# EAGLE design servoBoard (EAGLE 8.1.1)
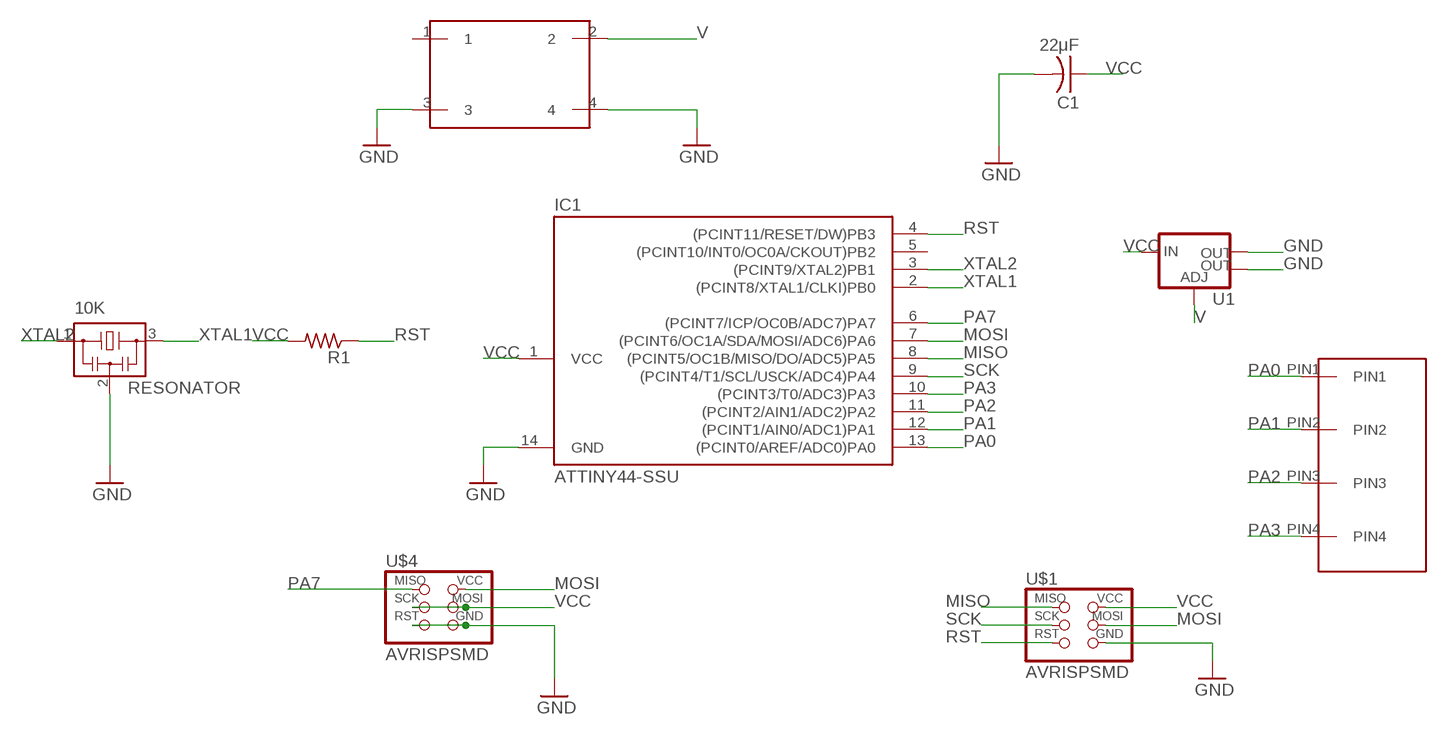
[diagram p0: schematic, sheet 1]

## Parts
10K  RESONATOR  [EFOBM]
C1  22μF  CAP-US1206FAB  [C1206FAB]
IC1  ATTINY44-SSU  [SOIC14]
R1  RES-US1206FAB  [R1206FAB]
U1  V_REG_LM1117SOT223  [SOT223]
U$1  AVRISPSMD  [2X03SMD]
U$2  4PINHEADER2X2  [2X02SMD]
U$3  4PINHEADER_ALTERNATE  [4PINHEADER]
U$4  AVRISPSMD  [2X03SMD]

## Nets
GND: 10K.2 C1.2 IC1.14(GND) U1.2(OUT) U1.4(OUT) U$1.6(GND) U$2.3 U$2.4 U$4.5(RST) U$4.6(GND)
MISO: IC1.8((PCINT5/OC1B/MISO/DO/ADC5)PA5) U$1.1(MISO)
MOSI: IC1.7((PCINT6/OC1A/SDA/MOSI/ADC6)PA6) U$1.4(MOSI) U$4.2(VCC)
PA0: IC1.13((PCINT0/AREF/ADC0)PA0) U$3.PIN1
PA1: IC1.12((PCINT1/AIN0/ADC1)PA1) U$3.PIN2
PA2: IC1.11((PCINT2/AIN1/ADC2)PA2) U$3.PIN3
PA3: IC1.10((PCINT3/T0/ADC3)PA3) U$3.PIN4
PA7: IC1.6((PCINT7/ICP/OC0B/ADC7)PA7) U$4.1(MISO)
RST: IC1.4((PCINT11/RESET/DW)PB3) R1.1 U$1.5(RST)
SCK: IC1.9((PCINT4/T1/SCL/USCK/ADC4)PA4) U$1.3(SCK)
V: U1.1(ADJ) U$2.2
VCC: C1.1 IC1.1(VCC) R1.2 U1.3(IN) U$1.2(VCC) U$4.3(SCK) U$4.4(MOSI)
XTAL1: 10K.3 IC1.2((PCINT8/XTAL1/CLKI)PB0)
XTAL2: 10K.1 IC1.3((PCINT9/XTAL2)PB1)
Unconnected: IC1.5((PCINT10/INT0/OC0A/CKOUT)PB2) U$2.1

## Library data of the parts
10K = fab:RESONATOR
C1 = fab:CAP-US
IC1 = fab:ATTINY44
R1 = fab:RES-US: Resistor (US Symbol)
U1 = fab:V_REG_LM1117: Voltage Regulator LM1117 Standard adjustable voltage regulator but in SMD form. Spark Fun Electronics SKU : COM-00595; PROD_ID: VREG-08170
U$1 U$4 = fab:AVRISP
U$2 = 4pinHeader2X2:4PINHEADER2X2
U$3 = 4pinHeaderAlternate:4PINHEADER_ALTERNATE

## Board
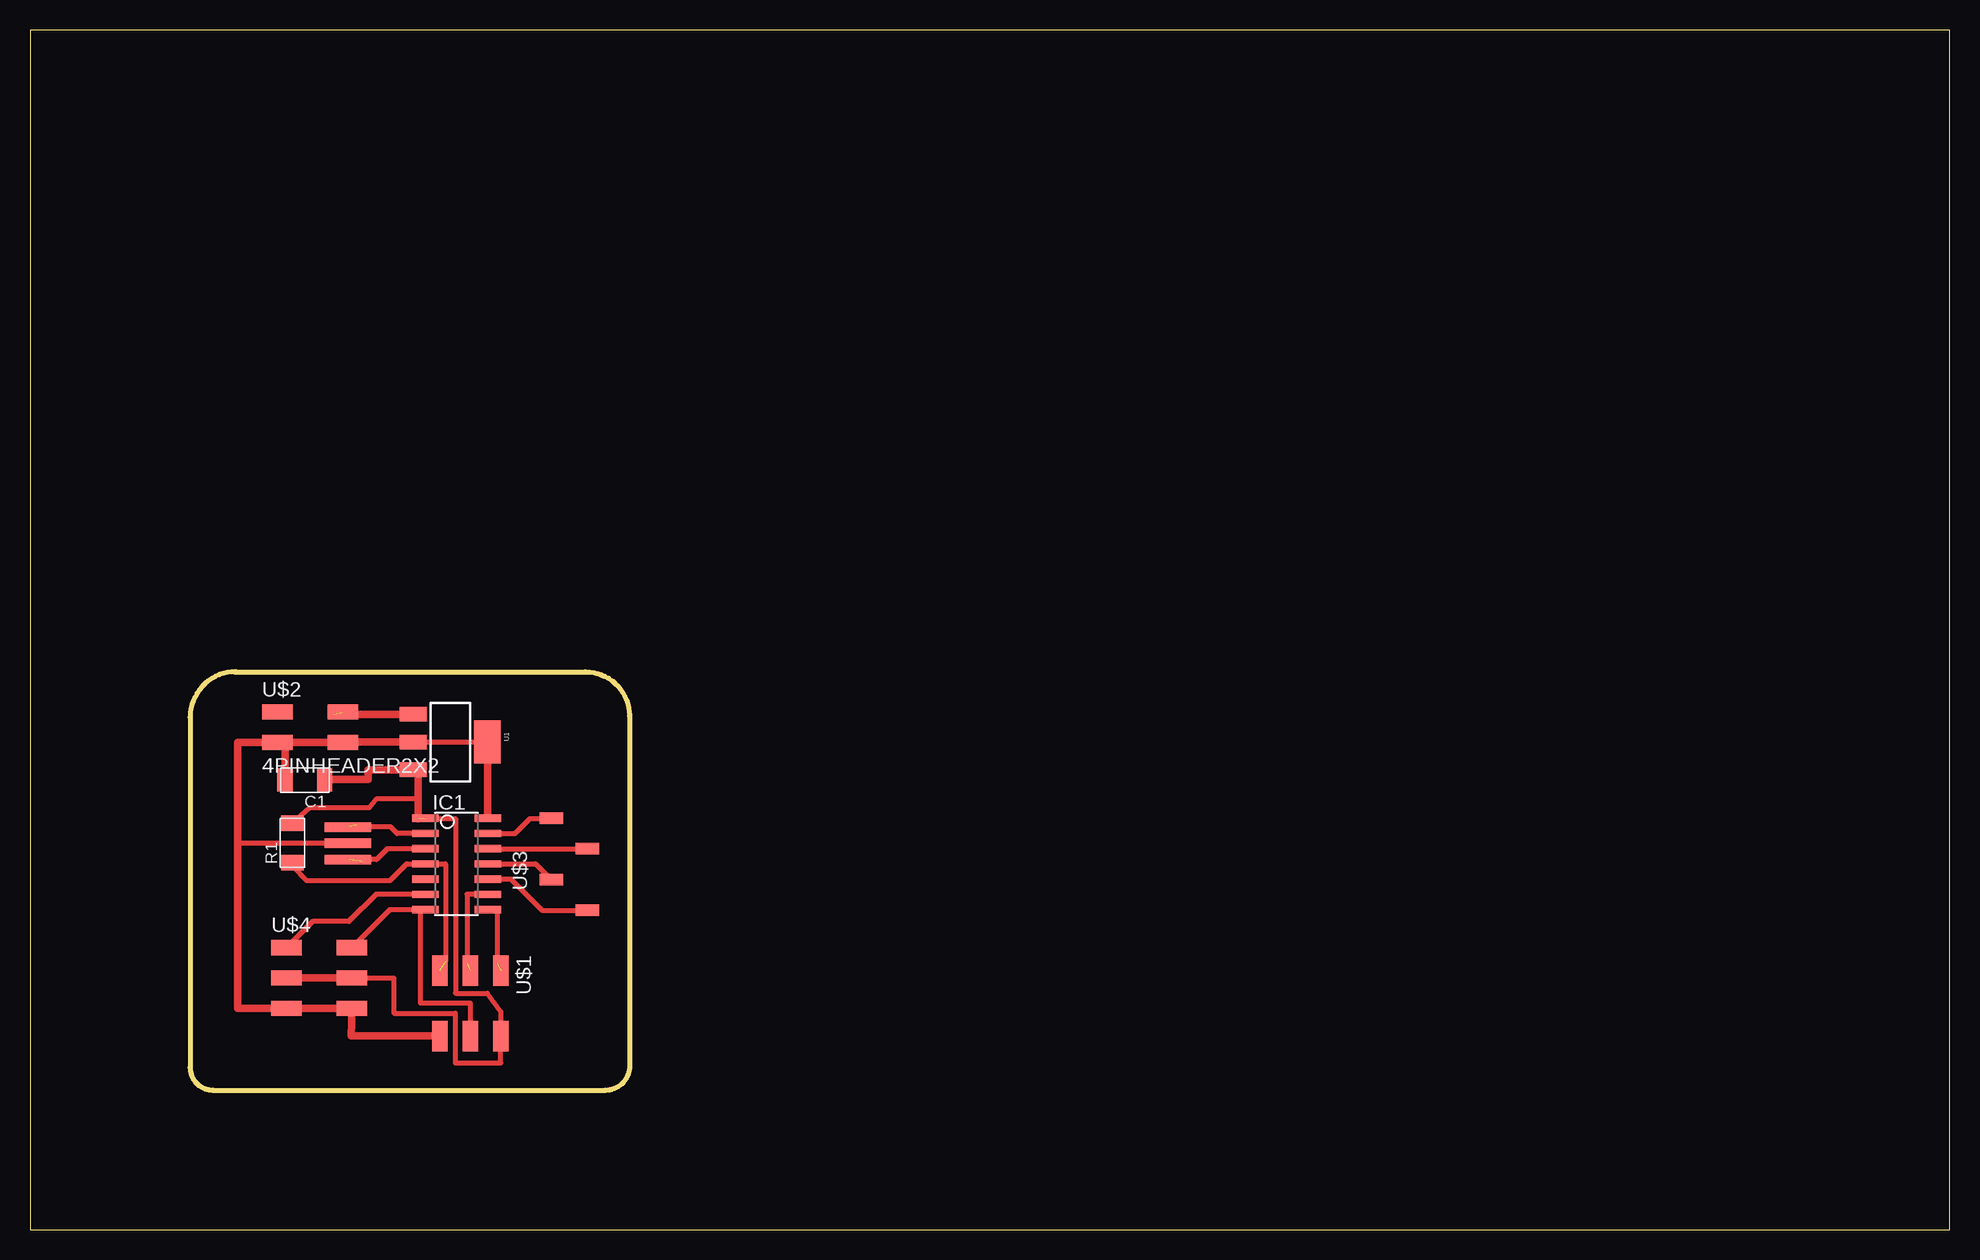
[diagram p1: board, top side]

Size 160 x 100 mm. Coordinates in mm from the lower left corner, seen from the top.
Outline: 17.01,46.49 46.31,46.49 arc-90 49.96,42.84
Outline: 17.17,46.51 arc90 13.35,42.69 13.35,13.5 arc90 15.23,11.62 47.97,11.62 arc90 50.01,13.66 50.01,42.94
Outline: 0,0 160,0 160,100 0,100 0,0
Copper layers (1*16): Top 0.035mm / dielectric 1.5mm / Bottom 0.035mm
Design rules "default": minimum track width 10mil, minimum drill 24mil, track to track 8mil, track to pad 8mil, pad to pad 8mil, via to via 8mil, smd to smd 8mil, copper to edge 40mil, drill to drill 8mil, minimum pad ring 10mil, minimum via ring 8mil, stop-mask expansion 4mil, vias tented up to drill 0mil, thermal gap 10mil

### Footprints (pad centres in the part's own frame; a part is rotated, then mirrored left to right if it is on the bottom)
EFOBM = smd 0.8 x 3.9: 1 -1.35,0; 2 0,0; 3 1.35,0
C1206FAB = smd 1.27 x 1.905: 1 -1.651,0; 2 1.651,0
SOIC14 = smd 0.61 x 2.21: 1 -3.81,-2.603; 2 -2.54,-2.603; 3 -1.27,-2.603; 4 0,-2.603; 5 1.27,-2.603; 6 2.54,-2.603; 7 3.81,-2.603; 8 3.81,2.603; 9 2.54,2.603; 10 1.27,2.603; 11 0,2.603; 12 -1.27,2.603; 13 -2.54,2.603; 14 -3.81,2.603
R1206FAB = smd 1.27 x 1.905: 1 -1.651,0; 2 1.651,0
SOT223 = smd 1.219 x 2.235: 1 -2.311,-3.099; 2 0,-3.099; 3 2.311,-3.099 | smd 3.6 x 2.2: 4 0,3.099
2X03SMD = smd 2.54 x 1.27: 1 -2.54,2.54; 2 2.92,2.54; 3 -2.54,0; 4 2.92,0; 5 -2.54,-2.54; 6 2.92,-2.54
2X02SMD = smd 2.54 x 1.27: 1 -2.54,1.27; 2 2.92,1.27; 3 -2.54,-1.27; 4 2.92,-1.27
4PINHEADER = smd 1.93 x 0.965: PIN1 0,0; PIN2 3,-2.54; PIN3 0,-5.12; PIN4 3,-7.66

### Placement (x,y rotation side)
10K  26.5,32.2 90 top
C1  22.91,37.47 180 top
IC1  35.56,30.48 270 top
R1  21.88,32.23 90 top
U1  35.04,40.64 270 top
U$1  36.7,19.06 270 top
U$2  23.15,41.87 0 top
U$3  43.46,34.28 0 top
U$4  23.93,20.97 0 top

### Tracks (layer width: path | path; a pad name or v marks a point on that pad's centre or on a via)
GND
  Top 0.406: 17.31,31.38 17.31,31.56 17.31,31.68 | 10K.2 17.31,32.2 17.31,32.53 | U1.2 U1.4
  Top 0.61: U1.4 38.16,40.64 IC1.14 | U1.2 26.07,40.64 U$2.4 20.09,40.6 20.09,40.61 | U$1.6 26.76,16.13 U$4.6 U$4.5 17.31,18.43 17.31,31.56 17.31,32.53 17.31,40.61 20.09,40.61 | 20.09,40.61 U$2.3 21.26,40.6 C1.2
MISO  (1 unrouted)
  Top 0.406: IC1.8 38.95,26.67 38.95,22.25
  Top 0.61: 38.39,26.67 IC1.8
MOSI
  Top 0.406: U$4.2 30.01,26.67 IC1.7 32.53,26.67 32.53,18.89 36.7,18.89 U$1.4
PA0
  Top 0.406: IC1.13 40.42,33.02 41.67,34.27 U$3.PIN1
PA1
  Top 0.406: IC1.12 U$3.PIN2
PA2
  Top 0.406: IC1.11 42.14,30.48 U$3.PIN3
PA3
  Top 0.406: IC1.10 40.07,29.21 42.67,26.61 U$3.PIN4
PA7
  Top 0.406: IC1.6 28.85,27.94 26.58,25.67 23.55,25.67 U$4.1
RST  (1 unrouted)
  Top 0.406: 34.64,22.37 34.64,30.48 IC1.4 31.4,30.48 30.02,29.1 23.04,29.1 21.88,30.26 R1.1
SCK  (1 unrouted)
  Top 0.406: IC1.9 36.42,27.94 36.42,22.2
V  (1 unrouted)
  Top 0.61: U1.1 25.3,42.95 25.3,43.09
VCC  (1 unrouted)
  Top 0.406: U$1.2 38.81,16.16 | IC1.1 32.96,34.27 35.46,34.27 35.47,19.69 38.12,19.69 39.24,18.15 U$1.2 | U$4.4 30.33,20.97 30.33,18.04 35.44,18.04 35.44,13.88 39.24,13.88 U$1.2 | 32.34,35.89 28.87,35.89 28.28,35.16 23.3,35.16 R1.2
  Top 0.61: U$4.3 U$4.4 | C1.1 24.56,37.53 28.18,37.53 28.18,38.33 U1.3 32.34,38.33 32.34,35.89 32.34,34.24
XTAL1  (1 unrouted)
  Top 0.406: IC1.2 30.6,33.02 30.05,33.57 27.35,33.57 27.21,33.71
XTAL2  (1 unrouted)
  Top 0.406: IC1.3 29.79,31.75 28.88,30.84 27.85,30.84 27.7,30.69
